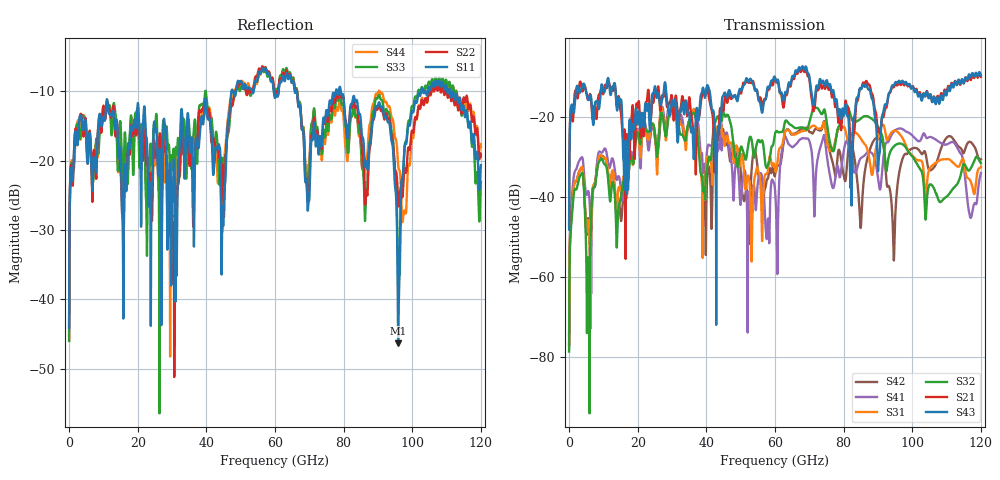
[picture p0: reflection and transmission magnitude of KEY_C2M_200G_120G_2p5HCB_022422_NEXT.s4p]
! Touchstone file
!  Generated:  9:03:34 AM  Nov 09, 2021
!  Setup:  LinearFrequency
!  Solution:  LinearFrequency
# GHz S MA R 50.000000
! Terminal data exported
! Port[1] = P2
! Port[2] = P4
! Port[3] = P6
! Port[4] = P8
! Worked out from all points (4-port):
!   12000 points, 10 MHz to 120 GHz, reference 50 ohm
!   strongest paths, dB at 10 MHz, 30.01 GHz, 60.01 GHz, 90.01 GHz, 120 GHz:
!     S43: -48.1, -15.8, -10.2, -33.5, -9.5
!     S21: -47.0, -15.0, -10.1, -23.6, -9.9
!     S32: -78.7, -18.0, -24.2, -22.4, -31.5
!     S31: -77.0, -16.7, -33.1, -25.0, -32.4
!     S41: -74.5, -16.7, -38.2, -35.2, -34.0
!     S42: -76.9, -17.5, -34.6, -25.2, -30.6
!   lowest |S11| = -46.3 dB at 95.88 GHz (marker M1), VSWR 1.01, Z = 50 + j0.483 ohm
!   |S11| at or under -10 dB: start of sweep to 47.3 GHz; 66.37 GHz to 77.71 GHz (11.34 GHz wide, 15.7 % of centre); 79.18 GHz to 102.6 GHz (23.41 GHz wide, 25.8 % of centre)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
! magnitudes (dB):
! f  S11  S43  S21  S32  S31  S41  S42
! 10 MHz  -44.1  -48.1  -47.0  -78.7  -77.0  -74.5  -76.9
! 3.13 GHz  -13.6  -13.9  -11.3  -34.9  -33.3  -30.7  -33.3
! 5.58 GHz  -19.1  -15.7  -15.5  -55.1  -45.7  -38.5  -45.3
! 30.19 GHz  -26.0  -16.1  -17.2  -18.4  -17.2  -16.5  -17.4
! 57.82 GHz  -7.5  -12.6  -13.2  -32.3  -33.9  -47.0  -35.5
! 95.88 GHz  -46.3  -11.2  -11.8  -26.7  -23.8  -22.9  -35.7
! 120 GHz  -20.6  -9.5  -9.9  -31.5  -32.4  -34.0  -30.6
